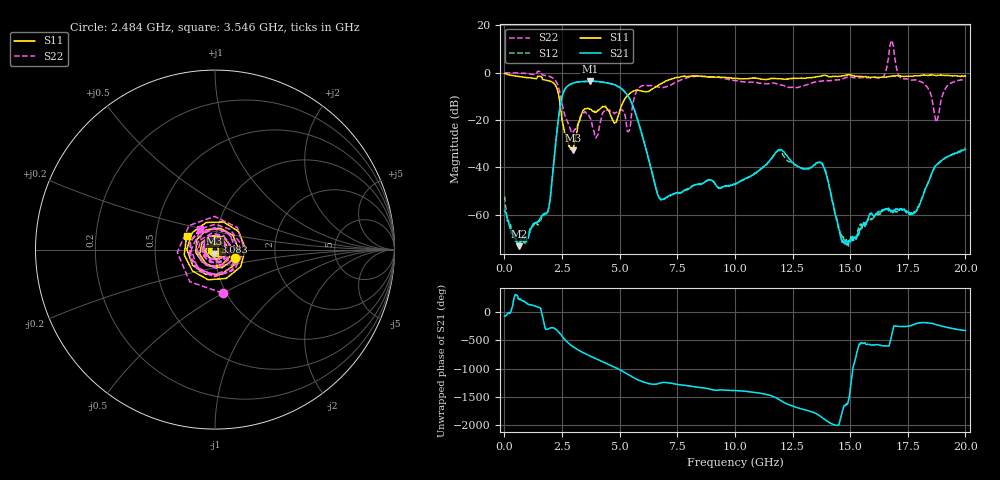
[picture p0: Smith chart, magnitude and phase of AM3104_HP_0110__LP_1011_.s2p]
!Created with skrf (http://scikit-rf.org).
# Hz S RI R 50.0
!freq ReS11 ImS11 ReS21 ImS21 ReS12 ImS12 ReS22 ImS22
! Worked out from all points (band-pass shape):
!   1601 points, 10 MHz to 20 GHz, reference 50 ohm
!   highest |S21| = -3.58 dB at 3.708 GHz (marker M1); lowest = -73.3 dB at 622.2 MHz (marker M2)
!   |S21| within 3 dB of the highest: 2.655 GHz to 5.053 GHz (2.398 GHz wide, 62.2 % of centre)
!   lowest |S11| = -32.8 dB at 2.971 GHz (marker M3), VSWR 1.05, Z = 49.6 - j2.24 ohm
!   |S11| at or under -10 dB: 2.365 GHz to 5.306 GHz (2.941 GHz wide, 76.7 % of centre)
!   |S22| runs from -27.6 to 13.6 dB; largest |S21 - S12| = 0.054
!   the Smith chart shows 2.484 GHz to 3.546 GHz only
!   S11 on the Smith chart (normalised r, x): 2.484 GHz: 1.25, -0.12; 3.083 GHz: 0.99, +0.08; 3.546 GHz: 0.72, +0.11
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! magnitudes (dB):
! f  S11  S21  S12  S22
! 10 MHz  -0.3  -58.3  -52.3  -0.1
! 622.2 MHz  -1.6  -73.3  -72.1  -0.2
! 1.884 GHz  -3.3  -58.6  -58.9  -1.4
! 2.484 GHz  -18.3  -10.9  -11.0  -12.2
! 2.971 GHz  -32.8  -4.4  -4.4  -25.2
! 3.083 GHz  -27.8  -4.1  -4.1  -23.9
! 3.346 GHz  -17.5  -3.8  -3.9  -17.8
! 3.546 GHz  -15.2  -3.7  -3.7  -17.0
! 3.708 GHz  -15.4  -3.6  -3.6  -19.0
! 4.795 GHz  -21.1  -5.1  -5.2  -17.2
! 5.382 GHz  -9.3  -10.1  -10.1  -24.9
! 5.807 GHz  -7.4  -20.8  -20.8  -6.8
! 6.682 GHz  -5.3  -52.3  -52.0  -6.1
! 10.01 GHz  -2.5  -47.3  -47.2  -3.4
! 11.93 GHz  -2.5  -32.5  -32.9  -5.0
! 13.34 GHz  -2.1  -39.9  -39.9  -4.4
! 13.87 GHz  -1.1  -40.1  -39.7  -3.3
! 14.72 GHz  -1.3  -71.7  -69.5  -2.5
! 16.68 GHz  -1.6  -57.6  -58.4  7.3
! 17.81 GHz  -1.3  -59.1  -59.1  -3.0
! 18.75 GHz  -1.2  -38.9  -39.1  -20.8
! 20 GHz  -1.4  -32.5  -31.8  -2.6
